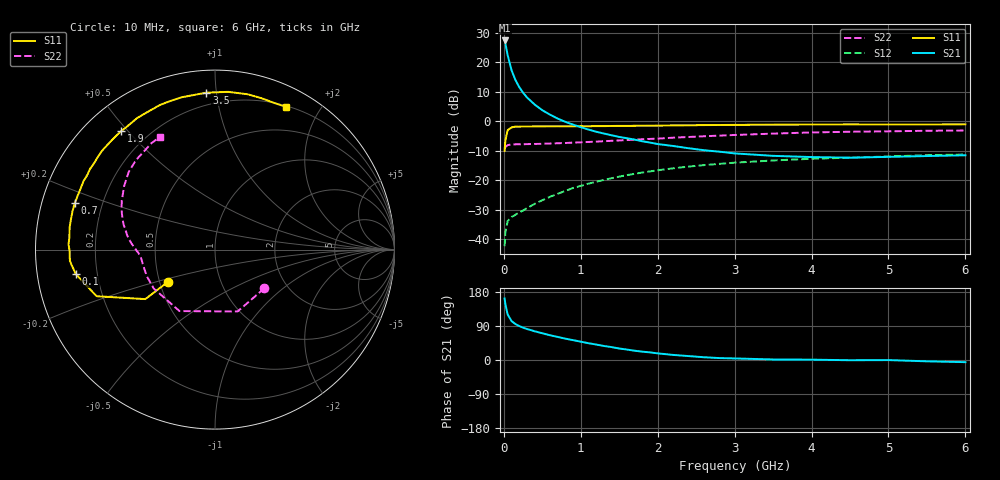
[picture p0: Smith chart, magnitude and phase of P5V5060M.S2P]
! SIEMENS Small Signal Semiconductors
! BFP183
! Si NPN RF Bipolar Junction Transistor in SOT143
! VCE = 0.5 V  IC = 60 mA
! Common Emitter S-Parameters:  March  1996
# GHz  S  MA  R  50
!  f  S11  S21  S12  S22
! GHz  MAG  ANG  MAG  ANG  MAG  ANG  MAG  ANG
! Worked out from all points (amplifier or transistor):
!   36 points, 10 MHz to 6 GHz, reference 50 ohm
!   highest |S21| = 27.4 dB at 10 MHz (marker M1)
!   |S21| within 3 dB of that: start of sweep to 34.98 MHz
!   unconditionally stable (mu >= 1): start of sweep to 37.61 MHz; 100.8 MHz to end of sweep
!   at 250 MHz: K = 1.66, MAG = 15.2 dB, |S12| = -30.2 dB
!   at 1.4 GHz: K = 2.18, MAG = 1.1 dB, |S12| = -19.3 dB
!   at 6 GHz: K = 1.39, MAG = -3.9 dB, |S12| = -11.3 dB
!   S11 on the Smith chart (normalised r, x): 10 MHz: 0.55, -0.22; 100 MHz: 0.12, -0.09; 700 MHz: 0.10, +0.16; 1.9 GHz: 0.11, +0.48; 3.5 GHz: 0.13, +0.94; 6 GHz: 0.21, +1.60
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0.01  0.3167 -145.6  23.32 162.2  0.0077 55.9  0.3495 -38.1
0.02  0.476 -144.6  20.82 146.8  0.0133 51.8  0.367 -69.9
0.05  0.7088 -158.5  13.08 119.9  0.0205 38.9  0.3955 -120.0
0.1  0.7878 -170.1  7.333 102.8  0.024 30.7  0.4044 -147.6
0.15  0.8111 -175.5  5.015 94.9  0.0261 34.4  0.4076 -158.4
0.2  0.8098 -179.3  3.791 89.6  0.0287 38.2  0.4077 -163.7
0.25  0.8169 177.9  3.047 85.4  0.0309 41.2  0.4086 -167.0
0.3  0.8142 175.5  2.54 81.9  0.0338 44.2  0.4107 -169.4
0.4  0.8192 171.4  1.922 75.8  0.0399 49.9  0.413 -172.2
0.5  0.8203 168.2  1.539 70.6  0.0461 52.0  0.4158 -174.0
0.6  0.8222 164.9  1.295 65.3  0.0527 54.4  0.4201 -175.6
0.7  0.8231 161.5  1.111 60.9  0.0593 55.7  0.4247 -176.9
0.9  0.8222 155.9  0.877 52.4  0.0743 56.2  0.4355 -178.8
1.1  0.8239 149.8  0.725 44.3  0.088 55.6  0.4466 179.1
1.5  0.836 139.1  0.543 30.3  0.1157 52.0  0.4738 174.5
1.9  0.8419 128.3  0.436 20.1  0.1418 46.7  0.5029 169.1
2.2  0.8517 120.6  0.382 13.4  0.1599 42.5  0.5278 164.7
2.8  0.8648 106.4  0.306 5.1  0.1902 33.7  0.5713 155.6
3.5  0.8758 93.1  0.26 1.4  0.2172 24.2  0.6184 144.9
4.5  0.8844 78.2  0.242 -0.6  0.2422 12.3  0.6654 131.4
5.5  0.8811 67.9  0.258 -3.5  0.2666 2.6  0.6906 120.9
6  0.8884 63.5  0.266 -5.7  0.2736 -2.5  0.6984 116.2
